(* Logix 5000 AddOnInstructionDefinition export MAC_COM; software revision 33.00 *)

TYPE JVL_AXIS_MAC :   // Drive Data
STRUCT
   ActualMode : DINT;   // actual Mode
   ActualPosition : REAL;   // P_IST
   ActualVelocity : REAL;   // V_IST(16)
   ActualTorque : REAL;   // ACTUAL_TORQUE
   AxisStatusError : JVL_MAC_Status_Error;   // Holds an indication of which error that is detected
   Home_Mode : DINT;   // Homemode
   RequestedMode : DINT;   // requested Mode
   RequestedPosition : REAL;   // P_SOLL
   RequestedVelocity : REAL;   // V_SOLL
   RequestedAcceleration : REAL;   // A_SOLL
   GeneralCommand : DINT;
   CommandTorque : REAL;   // Requested Torque, T_SOLL
   ZeroSearchVelocity : REAL;   // Homing velocity
   ZeroSearchPosition : REAL;   // Homing position
   ZeroSearchTorque : DINT;   // Homing torque setpoint threshold value
   ZeroSearchTThreshold : DINT;   // Threshold for torque zerosearch trigger, usually 20% lower than running torque
   TravelConst : REAL;   // Factor to multiply P_IST and P_SOLL for scaling
   VelConst : REAL;   // Factor to multiply V_SOLL and V_IST to get scaled velocity value
   HomingType : DINT;   // Holds the reqested homingtype
   LoadFactor : DINT;   // Inertia ratio motor/load
   MotorType : DINT;   // MotorType configured. 0=No Selection 1=MAC50-141-A/K (old) 2=MAC50-141-F (new), MAC400, 402, 1500, 3000, 4500 (All Encoder variations) 3=MAC800 with incremental encoder 4=MAC800 with abs. encoder
   Configured : DINT;
   MSG_OutValue : DINT;   // Used in exp. output message to the motor
   MSG_InValue : DINT;   // Used in Exp. output message, to get value from motor
   MSG_OutInstance : DINT;   // Registernumber
   MSG_InInstance : DINT;   // Registernummer
   V_SOLL_CountsPerSample : REAL;
   A_SOLL_CountsPerSample2 : REAL;
   AOI_Type : DINT;   // MAC_Disable = 1, MAC_Home = 2, MAC_Jog = 3, MAC_Position = 4, MAC_Reset = 5, MAC_Stop = 6
   Position_AppType : REAL;   // calculated Position by Application Type
   MSG_Out_Execute : BOOL;   // Enable MSG_Out
   MSG_In_Execute : BOOL;   // Enable MSG_In
   ErrorReset : BOOL;
   MSG_Out_Busy : BOOL;
   MSG_In_Busy : BOOL;
   MSG_Out_Done : BOOL;
   MSG_In_Done : BOOL;
END_STRUCT
END_TYPE

TYPE JVL_MAC_Status_Error :   // Axis Faults Status
STRUCT
   Error : BOOL;
   InitialisationError : BOOL;
   FlashMemoryError : BOOL;
   STOError : BOOL;
   NotUsed_2 : BOOL;
   NotUsed_3 : BOOL;
   OUT1 : BOOL;
   OUT2 : BOOL;
   NotUsed : BOOL;
   ControlVoltageError : BOOL;
   ShortCircuitError : BOOL;
   MotorSupplyDetected : BOOL;
   MotorLocked : BOOL;
   CommsError : BOOL;
   CurrentLoopError : BOOL;
   ModbusSlaveError : BOOL;
   TemperatureError : BOOL;
   UndervoltageError : BOOL;
   UndervoltageDetect : BOOL;
   OvervoltageError : BOOL;
   OvercurrentError : BOOL;
   OverspeedError : BOOL;
   AllowExceedingOfSoftwareLimits : BOOL;
   EncoderError : BOOL;
   I2TError : BOOL;
   FollowingError : BOOL;
   FunctionError : BOOL;
   BreakingResistorOverTempError : BOOL;
   InPosition : BOOL;
   Accelerating : BOOL;
   Decelerating : BOOL;
   SoftwareLimitExceeded : BOOL;
END_STRUCT
END_TYPE

ADD_ON_INSTRUCTION MAC_COM   (* revision 1.0 *)
VAR_IN_OUT
   JVL_IN : AB:ETHERNET_MODULE_DINT_32Bytes:I:0; {required}
   JVL_OUT : AB:ETHERNET_MODULE_DINT_32Bytes:O:0; {required}
   MSG_IN : MESSAGE; {required}
   MSG_OUT : MESSAGE; {required}
   AXIS : JVL_AXIS_MAC; {required}
END_VAR
VAR_INPUT
   MotorType : DINT; {required}   // 1=MAC50-141-A/K (old) 2=MAC50-141-F (new), MAC400, 402, 1500, 3000, 4500 (All Encoder variations) 3=MAC800 with incremental encoder 4=MAC800 with abs. encoder
   TravelPerRev : REAL := 1.0; {required}   // Travel per Revolution. Exc. actuator w. 60mm/rev, then value=60
   GearRatio : REAL := 1.0; {required}   // Gear ratio if a gearbox is mounted. select 1 for none
   ApplicationType : DINT; {required}   // Application_Type - 0=none (counts) 1=linear 2=degree
END_VAR
VAR
   CountsPerRevolution : REAL; {access None}
   vel : INT; {access None}
   torque : INT; {access None}
END_VAR

ROUTINE Logic   (* structured text *)
   
   
   	//MAC050F-141F (new mini MAC), MAC400, MAC402, MAC1500-MAC4500
   	IF MotorType = 2 THEN
   	    AXIS.V_SOLL_CountsPerSample := 2.84;
   	    AXIS.A_SOLL_CountsPerSample2 := 0.003693;
   		CountsPerRevolution:= 8192.0;
   	//MAC800-MAC1200 incremental encoder
   	ELSIF MotorType = 3 THEN
   	    AXIS.V_SOLL_CountsPerSample := 2.77;
   	    AXIS.A_SOLL_CountsPerSample2 := 0.003606;
   		CountsPerRevolution:= 8000.0;
   	//MAC800-MAC1200 absolute encoder
   	ELSIF MotorType = 4 THEN
   	    AXIS.V_SOLL_CountsPerSample := 2.84;
   	    AXIS.A_SOLL_CountsPerSample2 := 0.003606;
   		CountsPerRevolution:= 8192.0;
   	//MAC050-141-A/K (old mini MAC)
   	ELSIF MotorType = 1 THEN
   	    AXIS.V_SOLL_CountsPerSample := 2.1;
   	    AXIS.A_SOLL_CountsPerSample2 := 0.004026;
   		CountsPerRevolution:= 4096.0;
   	ELSE
   	    AXIS.V_SOLL_CountsPerSample := 0.0;
   	    AXIS.A_SOLL_CountsPerSample2 := 0.0;
   	END_IF;
   
   	AXIS.MotorType := MotorType;
   
   	//counts
   	if ApplicationType = 0 then
   	AXIS.TravelConst := 1;
   	AXIS.VelConst:= AXIS.V_SOLL_CountsPerSample;
   	//linear
   	elsif ApplicationType = 1 then
   	AXIS.TravelConst :=(CountsPerRevolution * GearRatio) / TravelPerRev;
   	AXIS.VelConst:= AXIS.V_SOLL_CountsPerSample * 60 * GearRatio / TravelPerRev;
   	//360°
   	elsif ApplicationType = 2 then
   	AXIS.TravelConst :=(CountsPerRevolution * GearRatio) / 360;
   	AXIS.VelConst:= AXIS.V_SOLL_CountsPerSample * 60 * GearRatio / 360;
   	end_if;
   
   
   AXIS.ActualMode := JVL_IN.Data[0];
   AXIS.ActualPosition := JVL_IN.Data[1];
   //AXIS.ActualVelocity := JVL_IN.Data[2];
   //AXIS.ActualTorque := JVL_IN.Data[3];
   vel:=JVL_IN.Data[2];
   torque:=JVL_IN.Data[3];
   if MotorType=1 then
   
   AXIS.ActualVelocity := trunc(vel*7.63);
   AXIS.ActualTorque := trunc(torque * 0.293);
   else
   AXIS.ActualVelocity := trunc(vel/AXIS.VelConst);
   AXIS.ActualTorque := trunc(torque * 0.293);
   end_if;
   AXIS.Home_Mode := JVL_IN.Data[5];
   
   AXIS.Position_AppType:= (AXIS.ActualPosition/AXIS.TravelConst);
   AXIS.AxisStatusError.Error := JVL_IN.Data[4].24;
   AXIS.AxisStatusError.InitialisationError := JVL_IN.Data[4].25;
   AXIS.AxisStatusError.FlashMemoryError := JVL_IN.Data[4].26;
   AXIS.AxisStatusError.STOError := JVL_IN.Data[4].27;
   AXIS.AxisStatusError.NotUsed_2 := JVL_IN.Data[4].28;
   AXIS.AxisStatusError.NotUsed_3 := JVL_IN.Data[4].29;
   AXIS.AxisStatusError.OUT1 := JVL_IN.Data[4].30;
   AXIS.AxisStatusError.OUT2 := JVL_IN.Data[4].31;
   AXIS.AxisStatusError.NotUsed := JVL_IN.Data[4].16;
   AXIS.AxisStatusError.ControlVoltageError := JVL_IN.Data[4].17;
   AXIS.AxisStatusError.ShortCircuitError := JVL_IN.Data[4].18;
   AXIS.AxisStatusError.MotorSupplyDetected := JVL_IN.Data[4].19;
   AXIS.AxisStatusError.MotorLocked := JVL_IN.Data[4].20;
   AXIS.AxisStatusError.CommsError := JVL_IN.Data[4].21;
   AXIS.AxisStatusError.CurrentLoopError := JVL_IN.Data[4].22;
   AXIS.AxisStatusError.ModbusSlaveError := JVL_IN.Data[4].23;
   AXIS.AxisStatusError.TemperatureError := JVL_IN.Data[4].8;
   AXIS.AxisStatusError.UndervoltageError := JVL_IN.Data[4].9;
   AXIS.AxisStatusError.UndervoltageDetect := JVL_IN.Data[4].10;
   AXIS.AxisStatusError.OvervoltageError := JVL_IN.Data[4].11;
   AXIS.AxisStatusError.OvercurrentError := JVL_IN.Data[4].12;
   AXIS.AxisStatusError.OverspeedError := JVL_IN.Data[4].13;
   AXIS.AxisStatusError.AllowExceedingOfSoftwareLimits := JVL_IN.Data[4].14;
   AXIS.AxisStatusError.EncoderError := JVL_IN.Data[4].15;
   AXIS.AxisStatusError.I2TError := JVL_IN.Data[4].0;
   AXIS.AxisStatusError.FollowingError := JVL_IN.Data[4].1;
   AXIS.AxisStatusError.FunctionError := JVL_IN.Data[4].2;
   AXIS.AxisStatusError.BreakingResistorOverTempError := JVL_IN.Data[4].3;
   AXIS.AxisStatusError.InPosition := JVL_IN.Data[4].4;
   AXIS.AxisStatusError.Accelerating := JVL_IN.Data[4].5;
   AXIS.AxisStatusError.Decelerating := JVL_IN.Data[4].6;
   AXIS.AxisStatusError.SoftwareLimitExceeded := JVL_IN.Data[4].7;
   
   JVL_OUT.Data[0]:= AXIS.RequestedMode;
   //cop(AXIS.RequestedPosition,JVL_OUT.Data[1],4);
   JVL_OUT.Data[1]:= AXIS.RequestedPosition;
   //cop(AXIS.RequestedVelocity,JVL_OUT.Data[2],4);
   JVL_OUT.Data[2]:= AXIS.RequestedVelocity;
   JVL_OUT.Data[3]:= AXIS.RequestedAcceleration;
   JVL_OUT.Data[4]:= AXIS.GeneralCommand;
   
   AXIS.MSG_Out_Done:= MSG_OUT.DN;
   AXIS.MSG_Out_Busy:= MSG_OUT.EN;
   AXIS.MSG_In_Done:= MSG_IN.DN;
   AXIS.MSG_In_Busy:= MSG_IN.EN;
   
   MSG_OUT.Instance:= AXIS.MSG_OutInstance;
   MSG_IN.Instance:= AXIS.MSG_InInstance;
END_ROUTINE
END_ADD_ON_INSTRUCTION

ADD_ON_INSTRUCTION MAC_Disable   (* revision 1.0 *)
VAR_IN_OUT
   AXIS : JVL_AXIS_MAC; {required}
END_VAR
VAR_OUTPUT
   Busy : BOOL; {access Read Only, visible}
   CommandAborted : BOOL; {access Read Only, visible}
   Done : BOOL; {access Read Only, visible}
   Error : BOOL; {access Read Only, visible}
END_VAR
VAR_INPUT
   Execute : BOOL; {required}
END_VAR
VAR
   State : INT; {access None}
   ExecuteStart : BOOL; {access None}
   AOI_Type : DINT; {access None}
END_VAR

ROUTINE Logic   (* structured text *)
   	//REGION CAPTURE EDGES
   	    if Execute and not ExecuteStart then
   	    	ExecuteStart:=1;
   		elsif not Execute then
   			ExecuteStart:=0;
   		end_if;
   
   	//END_REGION
   
   	//REGION STATE CHANGES
   
   	    //Re-trigger sequence from start on rising edge
   
   	    //Command aborted
   	    IF AXIS.AOI_Type <> AOI_Type AND
   	        State <> 0 AND
   	        State <> 90 AND
   	        State <> 30 AND
   	        State <> 80
   	    THEN
   	        State := 80;
   	    END_IF;
   
   
   	    //Error if motor error while executing
   	    IF AXIS.AxisStatusError.Error AND
   	        State <> 0 AND
   	        State <> 90 AND
   	        State <> 20 AND
   	        State <> 80
   	    THEN
   	        State := 90;
   	    END_IF;
   
   	//END_REGION
   
   	//REGION STATE MACHINE
   
   	    CASE State OF
   
   	        0:        //Wait for rising edge on execute
   	            IF ExecuteStart THEN
   					AOI_Type:= 1;
   					AXIS.AOI_Type:= 1;
   	                State := 10;
   	            END_IF;
   
   	        10:     //Put JVL into passive state
   	            AXIS.RequestedMode:= 0;
   	            IF AXIS.ActualMode = 0 THEN
   	                State := 20;
   	            END_IF;
   
   	        20:        //Disable complete, reset to idle by setting execute false
   	            IF NOT Execute THEN
   	                State := 0;
   	            END_IF;
   
   	        80:     //Aborted by other command before completion
   	            IF NOT Execute THEN
   	                State := 0;
   	            END_IF;
   
   	        90:       //Error while disabling, reset to idle by setting execute false
   	            IF NOT Execute THEN
   	                State := 0;
   	            END_IF;
   
   	        ELSE
   	            State := 90;
   
   	    END_CASE;
   
   	//END_REGION
   
   	//REGION STATUS SIGNALS
   
   	    Done := State = 20;
   	    CommandAborted := State = 80;
   	    Error := State = 90;
   	    Busy := State <> 0 AND NOT Done AND NOT Error AND NOT CommandAborted;
   
   	//END_REGION
   
END_ROUTINE
END_ADD_ON_INSTRUCTION

ADD_ON_INSTRUCTION MAC_Home   (* revision 1.0 *)
VAR_IN_OUT
   Axis : JVL_AXIS_MAC; {required}
END_VAR
VAR_OUTPUT
   Busy : BOOL; {access Read Only, visible}
   CommandAborted : BOOL; {access Read Only, visible}
   Done : BOOL; {access Read Only, visible}
   Error : BOOL; {access Read Only, visible}
END_VAR
VAR_INPUT
   Execute : BOOL; {required}
   Mode : INT; {required}
   Position : REAL; {required}
   Velocity : REAL; {required}
   Acceleration : REAL; {required}
   Offset : REAL; {required}
   TorqueLimit : REAL; {required}
END_VAR
VAR
   State : INT; {access None}
   ActiveMode : INT; {access None}
   Mode0State : INT; {access None}
   Mode1State : INT; {access None}
   ActivePosition : REAL; {access None}
   ActiveVelocity : REAL; {access None}
   ActiveAcceleration : REAL; {access None}
   ActiveTorqueLimit : REAL; {access None}
   ActiveOffset : REAL; {access None}
   Mode2State : INT; {access None}
   Mode3State : INT; {access None}
   ExecuteStart : BOOL; {access None}
   Ton_wait : FBD_TIMER; {access None}
   AOI_Type : DINT; {access None}
END_VAR

ROUTINE Logic   (* structured text *)
   	//REGION CAPTURE EDGES
   	    if Execute and not ExecuteStart then
   	    	ExecuteStart:=1;
   		elsif not Execute then
   			ExecuteStart:=0;
   		end_if;
   
   	//END_REGION
   
   	//REGION STATE CHANGES
   
   	    //Re-trigger sequence from start on rising edge
   
   
   	    //Command aborted
   	    IF Axis.AOI_Type <> AOI_Type AND
   	        State <> 0 AND
   	        State <> 90 AND
   	        State <> 30 AND
   	        State <> 80
   	    THEN
   	        State := 80;
   	    END_IF;
   
   
   	    //Error if motor error while executing
   	    IF Axis.AxisStatusError.Error AND
   	        State <> 0 AND
   	        State <> 90 AND
   	        State <> 30 AND
   	        State <> 80
   	    THEN
   	        State := 90;
   	    END_IF;
   	//END_REGION
   
   	//REGION STATE MACHINE
   
   
   
   	    CASE State OF
   
   	        0:
   	            //Reset static values
   	            ActiveMode := 0;
   	            ActivePosition := 0;
   	            ActiveVelocity := 0;
   	            ActiveAcceleration := 0;
   	            ActiveTorqueLimit := 0;
   	            ActiveOffset := 0;
   
   	            //Reset mode states
   	            Mode0State := 0;
   	            Mode1State := 0;
   	            Mode2State := 0;
   	            Mode3State := 0;
   
   	            IF ExecuteStart THEN
   					//
   					AOI_Type:= 2;
   					Axis.AOI_Type:= 2;
   	                //
   					Axis.GeneralCommand := 0;
   	                ActiveMode := Mode;
   	                ActivePosition := Position * Axis.TravelConst;
   	                ActiveVelocity := (Velocity) * Axis.VelConst;// * Axis.Device.Config.V_SOLL_CountsPerSample);
   	                ActiveAcceleration := ABS(Acceleration) * Axis.A_SOLL_CountsPerSample2;
   	                //set Acceleration always >=1
   	                IF ActiveAcceleration < 1 THEN
   	                    ActiveAcceleration := 1;
   	                END_IF;
   
   	                ActiveTorqueLimit := TorqueLimit * 3.41;//1024=300%;341=100%
   	                ActiveOffset := Offset * Axis.TravelConst;
   
   	                State := 10;
   	            END_IF;
   
   	        10:
   	            // change to velocity mode with zero setpoint to ensure motor does not run off to current position when homed
   	            IF ActiveAcceleration < 1 THEN
   	                Axis.RequestedAcceleration := 1;
   	            ELSE
   	                Axis.RequestedAcceleration := ActiveAcceleration;
   	            END_IF;
   	            Axis.RequestedVelocity := 0;
   	            Axis.RequestedMode := 1;
   	            // change position setpoint to new home position
   	            Axis.RequestedPosition := ActivePosition;
   	            // reset register trigger
   	            Axis.MSG_Out_Execute := 0;
   	            Axis.MSG_In_Execute := 0;
   	            // start homing
   	            State := 20;
   
   	        20:
   	            CASE ActiveMode OF
   
   	                0:  // Set Home Position
   	                    CASE Mode0State OF
   	                        0:
   	                            if Axis.MotorType=1 then
   									Axis.MSG_OutInstance := 163;
   								else
   									Axis.MSG_OutInstance := 4;
   								end_if;
   	                            Axis.MSG_OutValue:=Position;
   	                            Axis.MSG_Out_Execute := 1;
   	                            Axis.GeneralCommand := 16#0;
   	                            IF Axis.MSG_Out_Busy AND NOT Axis.MSG_Out_Done THEN
   	                                Mode0State := 10;
   	                            END_IF;
   	                        10:
   	                            IF Axis.MSG_Out_Done THEN
   	                                Axis.MSG_Out_Execute := 0;
   	                                Mode0State := 20;
   	                            END_IF;
   	                        20:
   	                            Axis.GeneralCommand := 16#800000F7;//16#10000F7 also
   	                            IF ABS(Axis.ActualPosition - Position) < 50.0 THEN
   	                                Mode0State := 30;
   	                            END_IF;
   	                        30:
   	                            Axis.GeneralCommand := 16#0;
   	                            Mode0State := 50;
   	                        50:
   	                            State := 30;
   	                        ELSE
   	                            State := 90;
   	                    END_CASE;
   
   	                1:  // Home to Sensor (type 2, bidirectional)
   	                    CASE Mode1State OF
   	                       0:
   	                            // reset hominging done bit old MAC050-141A/K
   	                                IF Axis.MotorType <> 1 THEN
   	                                    Mode1State := 10;
   	                                ELSE
   		                            Axis.MSG_OutInstance := 168;
   		                            Axis.MSG_OutValue := 0;
   		                            Axis.MSG_Out_Execute := 1;
   			                            IF Axis.MSG_Out_Busy THEN
   			                                Mode1State := 5;
   			                            END_IF;
   	                                END_IF;
   	                        5:
   	                            //Ton_Wait(IN := Reg.Done,PT := t#1s);
   	                            IF Axis.MSG_Out_Done THEN
   	                                Axis.MSG_Out_Execute := 0;
   	                                Mode1State := 10;
   	                            END_IF;
   	                       10:
   	                            //Home to Sensor (type 2);set homemode=3584
   	                            Axis.MSG_OutInstance := 42;
   	                            Axis.MSG_OutValue:=3584;
   
   	                            Axis.MSG_Out_Execute := 1;
   	                            IF Axis.MSG_Out_Busy THEN
   	                                Mode1State := 15;
   	                            END_IF;
   	                       15:
   	                            IF Axis.MSG_Out_Done THEN
   	                                Axis.MSG_Out_Execute := 0;
   	                                Mode1State := 20;
   	                            END_IF;
   
   	                       20:
   	                            // set home position offset move distance
   	                            Axis.MSG_OutInstance := 38;
   	                            Axis.MSG_OutValue:=ActiveOffset;
   	                            Axis.MSG_Out_Execute := 1;
   	                            IF Axis.MSG_Out_Busy THEN
   	                                Mode1State := 30;
   	                            END_IF;
   	                        30:
   	                            IF Axis.MSG_Out_Done THEN
   	                                Axis.MSG_Out_Execute := 0;
   	                                Mode1State := 40;
   	                            END_IF;
   	                        40:
   	                            // set homing approach velocity
   	                            Axis.MSG_OutInstance := 40;
   	                            Axis.MSG_OutValue:=ActiveVelocity;// * Axis.Device.Config.V_SOLL_CountsPerSample
   	                            Axis.MSG_Out_Execute := 1;
   	                            IF Axis.MSG_Out_Busy THEN
   	                                Mode1State := 50;
   	                            END_IF;
   	                        50:
   	                            IF Axis.MSG_Out_Done THEN
   	                                Axis.MSG_Out_Execute := 0;
   	                                Mode1State := 60;
   	                            END_IF;
   	                        60:
   	                            // start homing mode
   	                            Axis.RequestedMode := 14;
   								if Axis.MotorType=1 then
   									Axis.RequestedVelocity := ActiveVelocity;
   								end_if;
   	                            // homing done-register 42 Homemode bit 16
   	                            IF Axis.Home_Mode < 65536 THEN
   	                                Mode1State := 70;
   	                            END_IF;
   	                        70:
   	                            IF Axis.Home_Mode > 65536 AND Axis.MotorType <> 1 THEN
   	                                Axis.RequestedVelocity := 0;
   	                                Axis.RequestedMode := 2;
   	                                Mode1State := 80;
   	                            ELSIF Axis.Home_Mode > 0 AND Axis.MotorType = 1 THEN
   	                                Axis.RequestedVelocity := 0;
   	                                Axis.RequestedMode := 2;
   	                                Mode1State := 80;
   	                            END_IF;
   	                        80:
   	                            State := 30;
   	                        ELSE
   	                            State := 90;
   	                    END_CASE;
   
   	                2:  // Home to Endstop (torque limit)
   	                    CASE Mode2State OF
   	                        0:
   	                            //Home to Endstop (torque limit);set homemode=3072
   								Axis.MSG_OutInstance := 42;
   	                            Axis.MSG_OutValue := 3072;
   	                            Axis.MSG_Out_Execute := 1;
   
   	                            IF Axis.MSG_Out_Busy THEN
   	                                Mode2State := 5;
   	                            END_IF;
   	                        5:
   	                            IF Axis.MSG_Out_Done THEN
   	                                Axis.MSG_Out_Execute := 0;
   	                                Mode2State := 10;
   	                            END_IF;
   	                        10:
   								Axis.MSG_OutInstance := 38;
   	                            Axis.MSG_OutValue := ActiveOffset;
   	                            Axis.MSG_Out_Execute := 1;
   
   	                            IF Axis.MSG_Out_Busy THEN
   	                                Mode2State := 15;
   	                            END_IF;
   	                        15:
   	                            IF Axis.MSG_Out_Done THEN
   	                                Axis.MSG_Out_Execute := 0;
   	                                Mode2State := 20;
   	                            END_IF;
   	                        20:
   								Axis.MSG_OutInstance := 40;
   	                            Axis.MSG_OutValue := ActiveVelocity;// * Axis.Device.Config.V_SOLL_CountsPerSample;
   	                            Axis.MSG_Out_Execute := 1;
   	                            IF Axis.MSG_Out_Busy THEN
   	                                Mode2State := 25;
   	                            END_IF;
   	                        25:
   	                            IF Axis.MSG_Out_Done THEN
   	                                Axis.MSG_Out_Execute := 0;
   	                                IF Axis.MotorType <> 1 THEN
   	                                    Mode2State := 34;
   	                                ELSE
   	                                    Mode2State := 30;
   	                                END_IF;
   	                            END_IF;
   	                        30:
   	                            // reset hominging done bit old MAC050-141A/K
   								Axis.MSG_OutInstance := 168;
   	                            Axis.MSG_OutValue := 0;
   	                            Axis.MSG_Out_Execute := 1;
   
   	                            IF Axis.MSG_Out_Busy THEN
   	                                Mode2State := 32;
   	                            END_IF;
   	                        32:
   
   	                            IF Axis.MSG_Out_Done THEN
   	                                Axis.MSG_Out_Execute := 0;
   	                                Mode2State := 34;
   	                            END_IF;
   	                        34:
   								Axis.MSG_OutInstance := 41;
   	                            Axis.MSG_OutValue := ActiveTorqueLimit;
   	                            Axis.MSG_Out_Execute := 1;
   
   	                            IF Axis.MSG_Out_Busy THEN
   	                                Mode2State := 37;
   	                            END_IF;
   	                        37:
   	                            IF Axis.MSG_Out_Done THEN
   	                                Axis.MSG_Out_Execute := 0;
   	                                Mode2State := 40;
   	                            END_IF;
   	                        40:
   	                            Axis.RequestedMode := 12;
   	                            // homing done-register 42 Homemode bit 16
   								if Axis.MotorType=1 then
   									Axis.RequestedVelocity := ActiveVelocity;
   								end_if;
   	                            IF Axis.Home_Mode < 65536 THEN
   	                                Mode2State := 45;
   	                            END_IF;
   	                        45:
   	                            IF Axis.Home_Mode > 65536 AND Axis.MotorType <> 1 THEN
   	                                Axis.RequestedVelocity := 0;
   	                                Axis.RequestedMode := 2;
   	                                Mode2State := 60;
   	                            ELSIF Axis.Home_Mode > 0 AND Axis.MotorType = 1 THEN
   	                                Axis.RequestedVelocity := 0;
   	                                Axis.RequestedMode := 2;
   	                                Mode2State := 60;
   	                            END_IF;
   
   	                        60:
   	                            State := 30;
   	                        ELSE
   	                            State := 90;
   	                    END_CASE;
   
   
   	                3:  // Set Absolute Multiturn-Encoder
   	                    CASE Mode3State OF
   	                        0:
   	                            Ton_wait.TimerEnable:= 0;
   								Ton_wait.Reset:= 0;
   								Ton_wait.ACC:=0;
   
   								//read Absolute Encoder
   								Axis.MSG_InInstance := 226;
   	                            Axis.MSG_In_Execute := 1;
   	                            Axis.GeneralCommand := 16#0;
   	                            IF Axis.MSG_In_Busy AND NOT Axis.MSG_In_Done THEN
   	                                Mode3State := 5;
   	                            END_IF;
   	                        5:
   	                            IF Axis.MSG_In_Done THEN
   	                                //Absolute Encoder Value
   	                                ActiveOffset := Axis.MSG_InValue;
   	                                Axis.MSG_In_Execute := 0;
   	                                Mode3State := 10;
   	                            END_IF;
   	                        10:
   	                            //read HW Setup, contains Motor direction Reg 39 Bit 7
   								Axis.MSG_InInstance := 39;
   	                            Axis.MSG_In_Execute := 1;
   	                            IF Axis.MSG_In_Busy AND NOT Axis.MSG_In_Done THEN
   	                                Mode3State := 15;
   	                            END_IF;
   	                        15:
   	                            IF Axis.MSG_In_Done THEN
   	                                //Motor direction (true=inverted)
   	                                IF Axis.MSG_InValue.7 THEN
   	                                    ActivePosition := -ActivePosition + ActiveOffset;
   	                                ELSE
   	                                    ActivePosition := ActivePosition - ActiveOffset;
   	                                END_IF;
   	                                Axis.MSG_In_Execute := 0;
   	                                Mode3State := 20;
   	                            END_IF;
   	                        20:
   	                            //Set Absolute Encoder Offset
   								Axis.MSG_OutInstance := 225;
   	                            Axis.MSG_OutValue := ActivePosition;
   	                            Axis.MSG_Out_Execute := 1;
   
   	                            IF Axis.MSG_Out_Busy THEN
   	                                Mode3State := 25;
   	                            END_IF;
   	                        25:
   	                            IF Axis.MSG_Out_Done THEN
   	                                Axis.MSG_Out_Execute := 0;
   	                                Mode3State := 30;
   	                            END_IF;
   	                        30:
   	                            Axis.GeneralCommand := 16#110;//Save into flash
   	                            Mode3State := 40;
   	                        40:
   
   								TONR(Ton_wait);
   
   								Ton_wait.PRE:=6000;
   								Ton_wait.TimerEnable:= Mode3State = 40;
   	                            IF Ton_wait.DN THEN
   	                            	Axis.GeneralCommand := 16#0;
   	                                Mode3State := 50;
   									Ton_wait.Reset:= 1;
   	                            END_IF;
   
   	                        50:
   	                            State := 30;
                               	Axis.GeneralCommand := 16#0;
   								Ton_wait.Reset:= 0;
   	                        ELSE
   	                            State := 90;
   	                    END_CASE;
   
   	            END_CASE;
   
   	        30:        //Home complete, reset to idle by setting execute false
   	            IF NOT Execute THEN
   	                State := 0;
   	            END_IF;
   
   	        80:     //Aborted by other command before completion
   	            IF NOT Execute THEN
   	                State := 0;
   	            END_IF;
   
   	        90:       //Error while disabling, reset to idle by setting execute false
   	            IF NOT Execute THEN
   	                State := 0;
   	            END_IF;
   
   	        ELSE
   	            State := 90;
   
   	    END_CASE;
   
   	//END_REGION
   
   	//REGION STATUS SIGNALS
   
   	    Done := State = 30;
   	    CommandAborted := State = 80;
   	    Error := State = 90;
   	    Busy := State <> 0 AND NOT Done AND NOT Error AND NOT CommandAborted;
   
   	//END_REGION
END_ROUTINE
END_ADD_ON_INSTRUCTION

ADD_ON_INSTRUCTION MAC_Jog   (* revision 1.0 *)
VAR_IN_OUT
   AXIS : JVL_AXIS_MAC; {required}
END_VAR
VAR_INPUT
   JogForwards : BOOL; {required}
   JogBackwards : BOOL; {required}
END_VAR
VAR_OUTPUT
   Busy : BOOL; {access Read Only, visible}
   CommandAborted : BOOL; {access Read Only, visible}
   AtVelocity : BOOL; {access Read Only, visible}
   Error : BOOL; {access Read Only, visible}
END_VAR
VAR_INPUT
   Acceleration : REAL; {required}
   Velocity : REAL; {required}
END_VAR
VAR
   ForwardStart : BOOL; {access None}
   BackwardStart : BOOL; {access None}
   State : INT; {access None}
   ActiveVelocity : REAL; {access None}
   ActiveAcceleration : REAL; {access None}
   AOI_Type : DINT; {access None}
END_VAR

ROUTINE Logic   (* structured text *)
   	//REGION CAPTURE EDGES
   	    if JogForwards and not ForwardStart then
   	    	ForwardStart:=1;
   	    elsif JogBackwards  and not BackwardStart then
   	    	BackwardStart:=1;
   		elsif not JogForwards and not JogBackwards then
   			ForwardStart:=0;
   	    	BackwardStart:=0;
   		end_if;
   
   	//END_REGION
   
   	//REGION STATE CHANGES
   
   	    //Re-trigger sequence from start on rising edge
   	    //Command aborted
   	    IF AXIS.AOI_Type <> AOI_Type AND
   	        State <> 0 AND
   	        State <> 90 AND
   	        State <> 80
   	    THEN
   	        State := 80;
   	    END_IF;
   
   
   
   	    //Error if motor error while executing
   	    IF AXIS.AxisStatusError.Error AND
   	        State <> 0 AND
   	        State <> 90 AND
   	        State <> 80
   	    THEN
   	        State := 90;
   	    END_IF;
   
   	//END_REGION
   
   	//REGION STATE MACHINE
   
   	    CASE State OF
   
   	        0:
   	            ActiveVelocity := 0;
   	            ActiveAcceleration := 0;
   
   	            IF ForwardStart OR BackwardStart THEN
   					AOI_Type:= 3;
   					AXIS.AOI_Type:= 3;
   	                AXIS.RequestedMode:= 1;
   	                ActiveAcceleration := ABS(Acceleration)* AXIS.A_SOLL_CountsPerSample2;
   	                //set Acceleration always >=1
   	                IF ActiveAcceleration < 1 THEN
   	                    ActiveAcceleration := 1;
   	                END_IF;
   	                IF JogForwards AND not JogBackwards THEN
   	                    ActiveVelocity := ABS(Velocity) * AXIS.VelConst;// * Axis.Device.Config.V_SOLL_CountsPerSample));
   	                    State := 10;
   	                ELSIF JogBackwards AND NOT JogForwards THEN
   	                    ActiveVelocity := -1.0 * ABS(Velocity)* AXIS.VelConst;// * Axis.Device.Config.V_SOLL_CountsPerSample));
   	                    State := 10;
   	                ELSE
   	                    State := 30;
   	                END_IF;
   
   	                State := 10;
   	            END_IF;
   
   	        10:
   	            IF AXIS.ActualMode = 1 THEN
   
   	                AXIS.RequestedAcceleration := ActiveAcceleration;
   	                AXIS.RequestedVelocity := ActiveVelocity;
   
   	                IF JogForwards AND NOT JogBackwards THEN
   	                    State := 20;
   	                ELSIF JogBackwards AND NOT JogForwards THEN
   	                    State := 25;
   	                ELSE
   	                    State := 30;
   	                END_IF;
   
   	            END_IF;
   
   	        20:
   	            IF AXIS.ActualMode = 1 THEN
   
   	                IF NOT (JogForwards and not JogBackwards) THEN
   	                    State := 30;
   	                END_IF;
   
   	            ELSE
   	                State := 80;
   	            END_IF;
   
   	        25:
   	            IF AXIS.ActualMode = 1 THEN
   
   	                IF NOT (JogBackwards AND NOT JogForwards) THEN
   	                    State := 30;
   	                END_IF;
   
   	            ELSE
   	                State := 80;
   	            END_IF;
   
   	        30:
   	            AXIS.RequestedMode := 1;
   	            AXIS.RequestedVelocity := 0.0;
   
   	            State := 40;
   
   	        40:
   	            IF AXIS.ActualMode = 1  THEN
   
   	                //If no motion then stop is complete
   	                IF ABS((AXIS.ActualVelocity)) <= 10.0 AND
   	                    //Axis.Telegram.Input.StatusWord.AtVelocity AND
   	                    NOT AXIS.AxisStatusError.Accelerating AND
   	                    NOT AXIS.AxisStatusError.Decelerating THEN
   	                    State := 0;
   	                END_IF;
   
   	            ELSE
   	                State := 80;
   	            END_IF;
   
   	        80:     //Aborted by other command before completion
   	            IF NOT JogForwards AND NOT JogBackwards THEN
   	                State := 0;
   	            END_IF;
   
   	        90:       //Error while jogging, reset to idle by setting jog inputs false
   	            IF NOT JogForwards AND NOT JogBackwards THEN
   	                State := 0;
   	            END_IF;
   
   	        ELSE
   	            State := 90;
   
   	    END_CASE;
   
   	//END_REGION
   
   	//REGION STATUS SIGNALS
   
   	    AtVelocity:=(State=20 or State = 25) AND
   	                      //Axis.Telegram.Input.StatusWord.AtVelocity AND
   	                      AXIS.RequestedVelocity <> 0.0 AND
   	                      NOT AXIS.AxisStatusError.Accelerating AND
   	                      NOT AXIS.AxisStatusError.Decelerating;
   	    CommandAborted := State = 80;
   	    Error := State = 90;
   	    Busy := State <> 0 AND NOT Error AND NOT CommandAborted;
   
   	//END_REGION
   
END_ROUTINE
END_ADD_ON_INSTRUCTION

ADD_ON_INSTRUCTION MAC_Position   (* revision 1.0 *)
VAR_IN_OUT
   Axis : JVL_AXIS_MAC; {required}
END_VAR
VAR_OUTPUT
   Busy : BOOL; {access Read Only, visible}
   CommandAborted : BOOL; {access Read Only, visible}
   Done : BOOL; {access Read Only, visible}
   Error : BOOL; {access Read Only, visible}
END_VAR
VAR_INPUT
   Execute : BOOL; {required}
   Velocity : REAL; {required}
   Acceleration : REAL; {required}
   AbsolutePositioning : BOOL; {required}
   Position : REAL; {required}
END_VAR
VAR
   State : INT; {access None}
   ExecuteStart : BOOL; {access None}
   ActiveAbsolute : BOOL; {access None}
   ActiveVelocity : REAL; {access None}
   ActiveAcceleration : REAL; {access None}
   ActiveTargetPosition : REAL; {access None}
   StartPosition : REAL; {access None}
   AOI_Type : DINT; {access None}
END_VAR

ROUTINE Logic   (* structured text *)
   	//REGION CAPTURE EDGES
   	    if Execute and not ExecuteStart then
   	    	ExecuteStart:=1;
   		elsif not Execute then
   			ExecuteStart:=0;
   		end_if;
   
   	//END_REGION
   
   	//REGION STATE CHANGES
   
   	    //Re-trigger sequence from start on rising edge
   
   
   	    //Command aborted
   	    IF Axis.AOI_Type <> AOI_Type AND
   	        State <> 0 AND
   	        State <> 90 AND
   	        State <> 30 AND
   	        State <> 80
   	    THEN
   	        State := 80;
   	    END_IF;
   
   
   	    //Error if motor error while executing
   	    IF Axis.AxisStatusError.Error AND
   	        State <> 0 AND
   	        State <> 90 AND
   	        State <> 30 AND
   	        State <> 80
   	    THEN
   	        State := 90;
   	    END_IF;
   	//END_REGION
   
   	//REGION STATE MACHINE
   
   	    CASE State OF
   
   	        0:
   	            ActiveVelocity := 0;
   	            ActiveAcceleration := 0;
   	            ActiveAbsolute := 0;
   	            ActiveTargetPosition := 0;
   
   	            IF ExecuteStart THEN
   					AOI_Type:= 4;
   					Axis.AOI_Type:= 4;
   	                Axis.RequestedMode := 2;
   	                StartPosition := Axis.ActualPosition;// *Axis.TravelConst;
   	                ActiveVelocity := ABS(Velocity) * Axis.VelConst;// * Axis.Device.Config.V_SOLL_CountsPerSample);
   	                ActiveAcceleration := ABS(Acceleration)* Axis.A_SOLL_CountsPerSample2;
   	                //set Acceleration always >=1
   	                IF ActiveAcceleration < 1.0 THEN
   	                    ActiveAcceleration := 1.0;
   	                END_IF;
   
   	                ActiveAbsolute := AbsolutePositioning;
   
   	                IF ActiveAbsolute THEN
   	                    ActiveTargetPosition := Position *Axis.TravelConst;
   	                ELSE
   	                    ActiveTargetPosition := Position *Axis.TravelConst+ StartPosition;
   	                END_IF;
   
   	                State := 10;
   	            END_IF;
   
   	        10:
   	            IF Axis.ActualMode = 2 THEN
   	                Axis.RequestedAcceleration := ActiveAcceleration;
   	                Axis.RequestedPosition := ActiveTargetPosition;
   	                Axis.RequestedVelocity := ActiveVelocity;
   
   					State := 20;
   					(*
   	                IF ContinuousUpdate THEN
   	                    State := 25;
   	                ELSE
   	                    State := 20;
   	                END_IF;
   	                *)
   	            END_IF;
   
   	        20:
   	            IF Axis.ActualMode = 2 AND
   	                Axis.RequestedPosition = ActiveTargetPosition AND
   	                Axis.RequestedVelocity = ActiveVelocity THEN
   
   	                //If taget reached then move is complete
   	                IF ABS(ActiveTargetPosition - Axis.ActualPosition) <= 5.0 AND
   	                    Axis.AxisStatusError.InPosition AND
   	                    NOT Axis.AxisStatusError.Accelerating AND
   	                    NOT Axis.AxisStatusError.Decelerating THEN
   	                    State := 30;
   	                END_IF;
   
   	            ELSE
   	                State := 80;
   	            END_IF;
   
   	        30:
   	            IF NOT Execute THEN
   	                State := 0;
   	            END_IF;
   	        (*
   	        25:
   	            IF Axis.Telegram.Input.OperatingMode = 2 AND
   	                Axis.Telegram.Output.VelocitySetpoint = DINT_TO_DWORD(ActiveVelocity) AND
   	                Axis.Telegram.Output.PositionSetpoint = DINT_TO_DWORD(ActiveTargetPosition) THEN
   
   	                IF Execute THEN
   
   	                    ActiveVelocity := LREAL_TO_DINT(ABS(Velocity) * Axis.Device.Config.V_SOLL_CountsPerSample);
   	                    ActiveAcceleration := LREAL_TO_DINT(ABS(Acceleration) * Axis.Device.Config.A_SOLL_CountsPerSample2);
   	                    //set Acceleration always >=1
   	                    IF ActiveAcceleration < 1 THEN
   	                        ActiveAcceleration := 1;
   	                    END_IF;
   	                    IF ActiveAbsolute THEN
   	                        ActiveTargetPosition := Position;
   	                    ELSE
   	                        ActiveTargetPosition := Position + StartPosition;
   	                    END_IF;
   
   	                    Axis.Telegram.Output.AccelerationSetpoint := ActiveAcceleration;
   	                    Axis.Telegram.Output.PositionSetpoint := ActiveTargetPosition;
   	                    Axis.Telegram.Output.VelocitySetpoint := ActiveVelocity;
   
   	                    //If taget reached then move is complete
   	                    IF ABS(DINT_TO_LREAL(ActiveTargetPosition - Axis.Telegram.Input.ActualPosition)) <= 5.0 AND
   	                        Axis.Telegram.Input.StatusError.InPosition AND
   	                        NOT Axis.Telegram.Input.StatusError.Accelerating AND
   	                        NOT Axis.Telegram.Input.StatusError.Decelerating THEN
   	                        State := 35;
   	                    END_IF;
   
   	                ELSE
   	                    State := 20;
   	                END_IF;
   
   	            ELSE
   	                State := 80;
   	            END_IF;
   
   	        35:
   	            IF Execute THEN
   
   	                IF ActiveAbsolute THEN
   	                    IF ActiveTargetPosition <> Position THEN
   	                        State := 20;
   	                    END_IF;
   	                ELSE
   	                    IF ActiveTargetPosition <> (Position + StartPosition) THEN
   	                        State := 25;
   	                    END_IF;
   	                END_IF;
   
   	            ELSE
   	                State := 0;
   	            END_IF;
   	        *)
   	        80:     //Aborted by other command before completion
   	            IF NOT Execute THEN
   	                State := 0;
   	            END_IF;
   
   	        90:       //Error, reset to idle by setting execute false
   	            IF NOT Execute THEN
   	                State := 0;
   	            END_IF;
   	            //Mode=Passiv
   	            Axis.RequestedMode := 0;
   	        ELSE
   	            State := 90;
   
   	    END_CASE;
   
   	//END_REGION
   
   	//REGION STATUS SIGNALS
   
   	    Done := State = 30 OR State = 35;
   	    CommandAborted := State = 80;
   	    Error := State = 90;
   	    Busy := State <> 0 AND NOT Done AND NOT Error AND NOT CommandAborted;
   
   	//END_REGION
END_ROUTINE
END_ADD_ON_INSTRUCTION

ADD_ON_INSTRUCTION MAC_Reset   (* revision 1.0 *)
VAR_IN_OUT
   AXIS : JVL_AXIS_MAC; {required}
END_VAR
VAR_OUTPUT
   Busy : BOOL; {access Read Only, visible}
   CommandAborted : BOOL; {access Read Only, visible}
   Done : BOOL; {access Read Only, visible}
END_VAR
VAR_INPUT
   Execute : BOOL; {required}
END_VAR
VAR
   State : INT; {access None}
   ExecuteStart : BOOL; {access None}
   AOI_Type : DINT; {access None}
END_VAR

ROUTINE Logic   (* structured text *)
   	//REGION CAPTURE EDGES
   	    if Execute and not ExecuteStart then
   	    	ExecuteStart:=1;
   		elsif not Execute then
   			ExecuteStart:=0;
   		end_if;
   
   	//END_REGION
   
   	//REGION STATE CHANGES
   
   	    //Re-trigger sequence from start on rising edge
   	    //Command aborted
   	    IF AXIS.AOI_Type <> AOI_Type AND
   	        State <> 0 AND
   	        State <> 90 AND
   	        State <> 30 AND
   	        State <> 80
   	    THEN
   	        State := 80;
   	    END_IF;
   
   
   	//END_REGION
   
   	//REGION STATE MACHINE
   
   	    CASE State OF
   
   	        0:
   	            IF ExecuteStart THEN
   					AOI_Type:= 5;
   					AXIS.AOI_Type:= 5;
   	                AXIS.GeneralCommand := 16#0;
   	                State := 10;
   	            END_IF;
   
   	        10:
   	            AXIS.RequestedMode := 0;
   	            AXIS.RequestedAcceleration := 0;
   	            AXIS.RequestedPosition := 0;
   	            AXIS.RequestedVelocity := 0;
   	            AXIS.GeneralCommand := 16#800000E1;
   	            IF NOT AXIS.AxisStatusError.Error and AXIS.MotorType<>1 THEN
   	                State := 20;
   	            elsIF not AXIS.AxisStatusError.I2TError
   				and NOT AXIS.AxisStatusError.FollowingError
   				and NOT AXIS.AxisStatusError.FunctionError
   				and NOT AXIS.AxisStatusError.BreakingResistorOverTempError
   				and NOT AXIS.AxisStatusError.SoftwareLimitExceeded
   				and NOT AXIS.AxisStatusError.TemperatureError
   				and NOT AXIS.AxisStatusError.OvervoltageError
   				and NOT AXIS.AxisStatusError.OvercurrentError
   				and NOT AXIS.AxisStatusError.EncoderError
   				and AXIS.MotorType = 1 THEN
   	                State := 20;
   	            END_IF;
   
   
   	        20:
   	            AXIS.GeneralCommand := 16#0;
   	            State := 30;
   
   	        30:        //reset complete, reset to idle by setting execute false
   	            AXIS.GeneralCommand := 16#0;
   	            IF NOT Execute THEN
   	                State := 0;
   	            END_IF;
   
   	        80:     //Aborted by other command before completion
   	            IF NOT Execute THEN
   	                State := 0;
   	            END_IF;
   
   	        90:       //Error while disabling, reset to idle by setting execute false
   	            IF NOT Execute THEN
   	                State := 0;
   	            END_IF;
   
   	        ELSE
   	            State := 90;
   
   	    END_CASE;
   
   	//END_REGION
   
   	//REGION STATUS SIGNALS
   
   	    Done := State = 30;
   	    CommandAborted := State = 80;
   	    Busy := State <> 0 AND NOT Done AND NOT CommandAborted;
   
   	//END_REGION
   
END_ROUTINE
END_ADD_ON_INSTRUCTION

ADD_ON_INSTRUCTION MAC_Stop   (* revision 1.0 *)
VAR_IN_OUT
   AXIS : JVL_AXIS_MAC; {required}
END_VAR
VAR_OUTPUT
   CommandAborted : BOOL; {access Read Only, visible}
   Busy : BOOL; {access Read Only, visible}
   Done : BOOL; {access Read Only, visible}
   Error : BOOL; {access Read Only, visible}
END_VAR
VAR_INPUT
   Deceleration : REAL; {required}
   Execute : BOOL; {required}
END_VAR
VAR
   State : INT; {access None}
   ExecuteStart : BOOL; {access None}
   ActiveDeceleration : DINT; {access None}
   AOI_Type : DINT; {access None}
END_VAR

ROUTINE Logic   (* structured text *)
   	//REGION CAPTURE EDGES
   	    if Execute and not ExecuteStart then
   	    	ExecuteStart:=1;
   		elsif not Execute then
   			ExecuteStart:=0;
   		end_if;
   
   	//END_REGION
   
   	//REGION STATE CHANGES
   
   	    //Re-trigger sequence from start on rising edge
   
   	    //Command aborted
   	    IF AXIS.AOI_Type <> AOI_Type AND
   	        State <> 0 AND
   	        State <> 90 AND
   	        State <> 30 AND
   	        State <> 80
   	    THEN
   	        State := 80;
   	    END_IF;
   
   	    //Error if motor error while executing
   	    IF AXIS.AxisStatusError.Error AND
   	        State <> 0 AND
   	        State <> 90 AND
   	        State <> 30 AND
   	        State <> 80
   	    THEN
   	        State := 90;
   	    END_IF;
   
   	//END_REGION
   
   	//REGION STATE MACHINE
   
   	    CASE State OF
   
   	        0:        //Wait for rising edge on execute
   	            ActiveDeceleration := 0;
   
   	            IF ExecuteStart THEN
   					AOI_Type:= 6;
   					AXIS.AOI_Type:= 6;
   	                AXIS.RequestedMode:= 1;
   	                ActiveDeceleration :=  Deceleration;// * Axis.Device.Config.A_SOLL_CountsPerSample2);
   	                //set Acceleration always >=1
   	                IF ActiveDeceleration < 1 THEN
   	                    ActiveDeceleration := 1;
   	                END_IF;
   	                State := 10;
   	            END_IF;
   
   	        10:        //Trigger stop
   	            IF AXIS.ActualMode = 1 THEN
   	                AXIS.RequestedAcceleration := ActiveDeceleration;
   	                AXIS.RequestedVelocity := 0.0;
   	                State := 20;
   
   	            ELSE            //Go to Idle if other command has changed the operating state
   	                State := 0;
   	            END_IF;
   
   	        20:    //Check stop is complete
   	            IF AXIS.RequestedMode = 1 AND
   	                AXIS.RequestedVelocity = 0 THEN
   
   	                //If no motion then stop is complete
   	                IF ABS(AXIS.ActualVelocity) <= 10.0 AND
   	                    NOT AXIS.AxisStatusError.Accelerating and
   	                    NOT AXIS.AxisStatusError.Decelerating THEN
   	                    State := 30;
   	                END_IF;
   
   	            ELSE            //Go to Idle if other command has changed the operating state
   	                State := 0;
   	            END_IF;
   
   	        30:        //Disable complete, reset to idle by setting execute false
   	            IF NOT Execute THEN
   	                State := 0;
   					ExecuteStart:=0;
   
   	            END_IF;
   
   	        80:     //Aborted by other command before completion
   	            IF NOT Execute THEN
   	                State := 0;
   					ExecuteStart:=0;
   	            END_IF;
   
   	        90:       //Error while disabling, reset to idle by setting execute false
   	            IF NOT Execute THEN
   	                State := 0;
   					ExecuteStart:=0;
   	            END_IF;
   
   	        ELSE
   	            State := 90;
   
   	    END_CASE;
   
   	//END_REGION
   
   	//REGION STATUS SIGNALS
   
   	    Done := State = 30;
   	    CommandAborted := State = 80;
   	    Error := State = 90;
   	    Busy := State <> 0 AND NOT Done AND NOT Error AND NOT CommandAborted;
   
   	//END_REGION
END_ROUTINE
END_ADD_ON_INSTRUCTION
